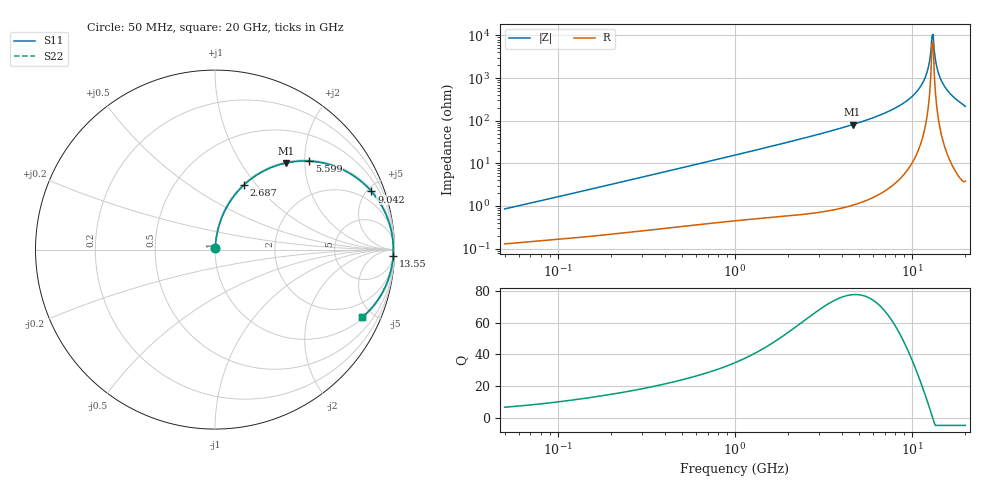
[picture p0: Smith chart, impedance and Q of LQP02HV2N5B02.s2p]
!Murata Part Number: LQP02HV2N5B02
!These Parameters are Measured in Series Mode Connection
!  o--[Z]--o
!Port1  Port2
!  o-------o
!Freq. Start=50[MHz] Stop=20[GHz], 401[Steps]
# Hz S RI R 50
!Freq.(Hz) S11(Real) S11(Imag) S21(Real) S21(Imag) S12(Real) S12(Imag) S22(Real) S22(Imag)
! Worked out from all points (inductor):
!   401 points, 50 MHz to 20 GHz, reference 50 ohm
!   read as one part in series: L = 2.66 nH near 51.52 MHz
!   highest Q = 77.7 at 4.608 GHz (marker M1), where L = 2.79 nH
!   self-resonance near 12.95 GHz
!   S11 on the Smith chart (normalised r, x): 50 MHz: 1.00, +0.02; 2.687 GHz: 1.01, +0.86; 5.599 GHz: 1.03, +2.11; 9.042 GHz: 1.11, +5.33; 13.55 GHz: 10, -53; 20 GHz: 1.08, -4.33
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5e7  0.00136 0.00842  0.9986 -0.00842  0.9986 -0.00842  0.00136 0.00842
1.364002e8  0.00235 0.022  0.9977 -0.022  0.9977 -0.022  0.00235 0.022
3.721004e8  0.0063 0.0583  0.9937 -0.0583  0.9937 -0.0583  0.0063 0.0583
1e9  0.028 0.1512  0.972 -0.1512  0.972 -0.1512  0.028 0.1512
2.687447e9  0.1612 0.36  0.8388 -0.36  0.8388 -0.36  0.1612 0.36
2.728004e9  0.1655 0.364  0.8345 -0.364  0.8345 -0.364  0.1655 0.364
4.608136e9  0.397 0.4829  0.603 -0.4829  0.603 -0.4829  0.397 0.4829
5.598765e9  0.526 0.4928  0.474 -0.4928  0.474 -0.4928  0.526 0.4928
7.442007e9  0.738 0.4319  0.262 -0.4319  0.262 -0.4319  0.738 0.4319
9.041845e9  0.8715 0.3242  0.1285 -0.3242  0.1285 -0.3242  0.8715 0.3242
1.034674e10  0.9418 0.2192  0.0582 -0.2192  0.0582 -0.2192  0.9418 0.2192
1.149051e10  0.9774 0.1243  0.0226 -0.1243  0.0226 -0.1243  0.9774 0.1243
1.220001e10  0.9889 0.0668  0.0111 -0.0668  0.0111 -0.0668  0.9889 0.0668
1.276073e10  0.993 0.0227  0.00701 -0.0227  0.00701 -0.0227  0.993 0.0227
1.295331e10  0.9935 0.00792  0.00651 -0.00792  0.00651 -0.00792  0.9935 0.00792
1.334722e10  0.9932 -0.0217  0.00685 0.0217  0.00685 0.0217  0.9932 -0.0217
1.354865e10  0.9923 -0.0364  0.00767 0.0364  0.00767 0.0364  0.9923 -0.0364
1.375312e10  0.9911 -0.0512  0.00894 0.0512  0.00894 0.0512  0.9911 -0.0512
1.417136e10  0.9872 -0.0805  0.0128 0.0805  0.0128 0.0805  0.9872 -0.0805
1.527346e10  0.97 -0.1522  0.03 0.1522  0.03 0.1522  0.97 -0.1522
1.721783e10  0.9214 -0.2586  0.0786 0.2586  0.0786 0.2586  0.9214 -0.2586
2e10  0.8202 -0.3753  0.1798 0.3753  0.1798 0.3753  0.8202 -0.3753
